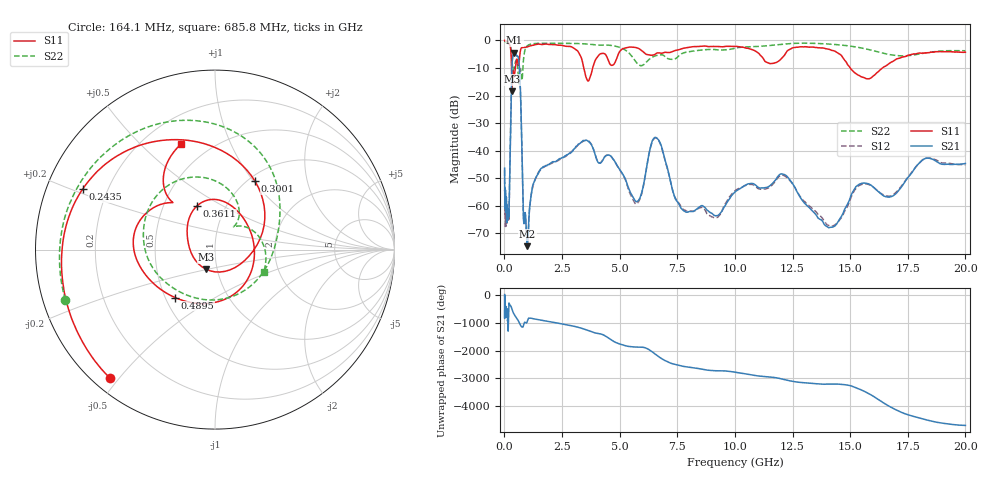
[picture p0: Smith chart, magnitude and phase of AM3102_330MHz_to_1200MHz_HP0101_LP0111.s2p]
! Date/Time: Tue, Sep 11, 2018 5:14 PM
! Network Analyzer: Agilent Technologies E8362B Rev: A.07.50.63
! Sweep from 0.010 to 20.000 GHz, 1601 Points, Sweep Type: LOG
! Power Supply: 4.949 V, 0.001 A
# Hz S DB R 50
!freq MagS11 AngS11 MagS21 AngS21 MagS12 AngS12 MagS22 AngS22
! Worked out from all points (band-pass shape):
!   1601 points, 10 MHz to 20 GHz, reference 50 ohm
!   highest |S21| = -4.48 dB at 434.6 MHz (marker M1); lowest = -74.7 dB at 998.1 MHz (marker M2)
!   |S21| within 3 dB of the highest: 341.3 MHz to 630 MHz (288.7 MHz wide, 59.4 % of centre)
!   lowest |S11| = -18.4 dB at 331.5 MHz (marker M3), VSWR 1.27, Z = 44.2 - j9.79 ohm
!   |S11| at or under -10 dB: 309.3 MHz to 476.9 MHz (167.6 MHz wide, 42.6 % of centre); 3.445 GHz to 3.828 GHz (383.8 MHz wide, 10.6 % of centre); 15.01 GHz to 16.4 GHz (1.398 GHz wide, 8.9 % of centre)
!   |S22| runs from -15.7 to -0.2 dB; largest |S21 - S12| = 0.01
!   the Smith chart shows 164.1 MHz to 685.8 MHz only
!   S11 on the Smith chart (normalised r, x): 164.1 MHz: 0.05, -0.47; 243.5 MHz: 0.11, +0.22; 300.1 MHz: 1.07, +1.02; 361.1 MHz: 0.73, +0.38; 489.5 MHz: 0.56, -0.34; 685.8 MHz: 0.35, +0.67
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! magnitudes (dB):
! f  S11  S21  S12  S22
! 10 MHz  0.0  -46.4  -47.2  -0.2
! 35.55 MHz  0.0  -59.8  -57.1  -0.4
! 126.4 MHz  -0.4  -65.1  -63.2  -0.9
! 164.1 MHz  -0.7  -62.6  -63.8  -1.1
! 243.5 MHz  -1.8  -44.4  -44.3  -1.8
! 300.1 MHz  -7.1  -17.9  -18.0  -3.8
! 331.5 MHz  -18.4  -8.8  -8.8  -7.7
! 361.1 MHz  -11.6  -6.0  -6.1  -10.6
! 434.6 MHz  -12.6  -4.5  -4.5  -9.3
! 447.2 MHz  -11.8  -4.5  -4.5  -8.8
! 489.5 MHz  -9.2  -4.8  -4.9  -7.5
! 685.8 MHz  -4.2  -15.8  -15.9  -10.5
! 829.3 MHz  -2.5  -64.8  -64.2  -7.0
! 998.1 MHz  -2.3  -74.7  -74.0  -1.9
! 1.59 GHz  -1.4  -46.5  -46.8  -1.0
! 3.582 GHz  -14.2  -36.3  -36.3  -1.3
! 5.652 GHz  -2.5  -58.0  -58.9  -7.1
! 6.549 GHz  -5.0  -35.2  -35.4  -5.6
! 9.047 GHz  -2.2  -63.1  -64.2  -3.2
! 12.09 GHz  -5.9  -48.6  -49.0  -1.3
! 14.14 GHz  -3.4  -67.9  -67.5  -1.3
! 20 GHz  -4.3  -44.7  -45.2  -3.7
